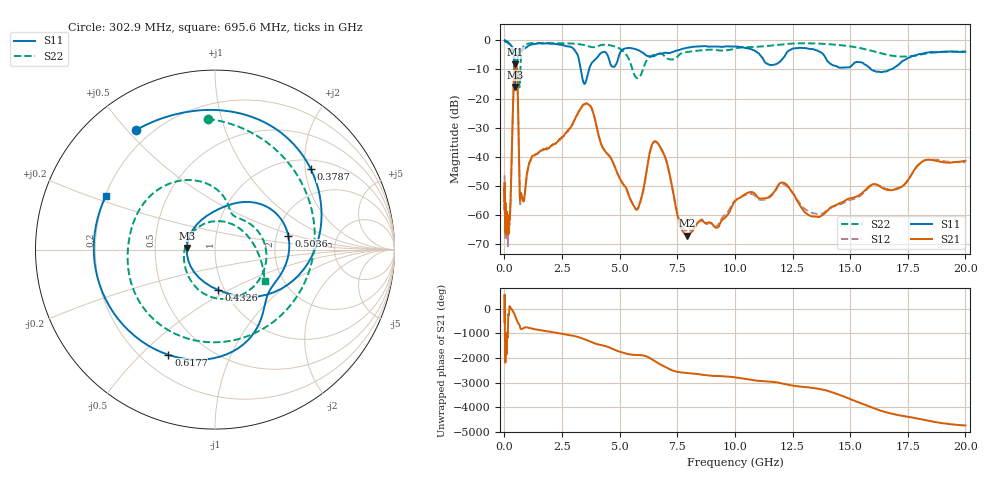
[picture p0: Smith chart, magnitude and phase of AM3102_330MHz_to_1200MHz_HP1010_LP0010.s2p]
! Date/Time: Tue, Sep 11, 2018 5:18 PM
! Network Analyzer: Agilent Technologies E8362B Rev: A.07.50.63
! Sweep from 0.010 to 20.000 GHz, 1601 Points, Sweep Type: LOG
! Power Supply: 4.949 V, 0.001 A
# Hz S DB R 50
!freq MagS11 AngS11 MagS21 AngS21 MagS12 AngS12 MagS22 AngS22
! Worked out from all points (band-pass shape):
!   1601 points, 10 MHz to 20 GHz, reference 50 ohm
!   highest |S21| = -8.26 dB at 475.7 MHz (marker M1); lowest = -67.2 dB at 7.92 GHz (marker M2)
!   |S21| within 3 dB of the highest: 424.2 MHz to 555.5 MHz (131.3 MHz wide, 26.8 % of centre)
!   lowest |S11| = -16.1 dB at 449.3 MHz (marker M3), VSWR 1.37, Z = 36.4 + j0.717 ohm
!   |S11| at or under -10 dB: 425.5 MHz to 476.3 MHz (50.85 MHz wide, 11.3 % of centre); 3.312 GHz to 3.669 GHz (356.7 MHz wide, 10.2 % of centre); 15.92 GHz to 16.76 GHz (841.7 MHz wide, 5.15 % of centre)
!   |S22| runs from -16.1 to -0.2 dB; largest |S21 - S12| = 0.0067
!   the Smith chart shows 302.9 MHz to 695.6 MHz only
!   S11 on the Smith chart (normalised r, x): 302.9 MHz: 0.14, +0.53; 378.7 MHz: 1.23, +2.14; 432.6 MHz: 0.94, -0.45; 503.6 MHz: 2.33, +0.43; 617.7 MHz: 0.31, -0.61; 695.6 MHz: 0.20, +0.22
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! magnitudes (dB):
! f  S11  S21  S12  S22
! 10 MHz  0.0  -51.2  -46.4  -0.2
! 35.55 MHz  0.0  -61.7  -63.6  -0.3
! 126.4 MHz  -0.4  -63.0  -66.0  -0.7
! 243.5 MHz  -1.2  -60.6  -59.7  -1.5
! 302.9 MHz  -2.0  -44.6  -44.6  -2.7
! 378.7 MHz  -3.1  -21.4  -21.4  -5.7
! 432.6 MHz  -12.9  -10.2  -10.2  -6.0
! 447.2 MHz  -16.0  -8.9  -8.9  -6.3
! 449.3 MHz  -16.1  -8.8  -8.8  -6.3
! 475.7 MHz  -10.1  -8.3  -8.4  -6.5
! 503.6 MHz  -7.6  -8.4  -8.4  -7.8
! 561.8 MHz  -7.4  -12.4  -12.5  -13.1
! 617.7 MHz  -3.9  -32.6  -32.6  -11.2
! 695.6 MHz  -3.4  -54.9  -55.9  -9.7
! 1.59 GHz  -1.0  -37.9  -37.9  -0.9
! 3.617 GHz  -11.7  -21.9  -21.7  -1.9
! 5.652 GHz  -2.9  -57.5  -57.7  -12.1
! 6.643 GHz  -4.7  -35.3  -35.3  -4.7
! 7.92 GHz  -2.5  -67.2  -65.6  -4.0
! 12.03 GHz  -6.6  -48.9  -49.4  -1.4
! 13.61 GHz  -3.7  -60.8  -59.7  -1.1
! 20 GHz  -3.9  -41.4  -42.0  -3.8
